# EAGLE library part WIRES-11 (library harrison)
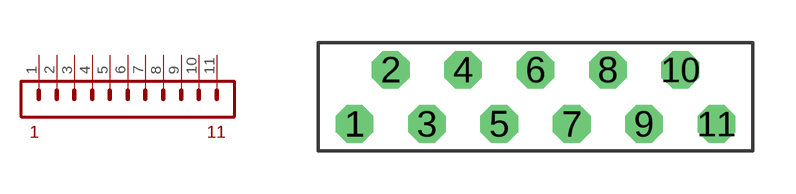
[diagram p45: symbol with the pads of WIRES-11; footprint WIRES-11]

Designator prefix -

## WIRES-11  [WIRES-11]
1  1  pas
2  2  pas
3  3  pas
4  4  pas
5  5  pas
6  6  pas
7  7  pas
8  8  pas
9  9  pas
10  10  pas
11  11  pas

## Footprint WIRES-11 (pad centres in mm)
drill 0.813 octagon: 1 -6.35,-0.635; 2 -5.08,1.27; 3 -3.81,-0.635; 4 -2.54,1.27; 5 -1.27,-0.635; 6 0,1.27; 7 1.27,-0.635; 8 2.54,1.27; 9 3.81,-0.635; 10 5.08,1.27; 11 6.35,-0.635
